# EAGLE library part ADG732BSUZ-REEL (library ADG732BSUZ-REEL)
16-/32-Channel, 4 , +1.8 V to +5.5 V and +/-2.5 V Analog Multiplexers. Source: Datasheet
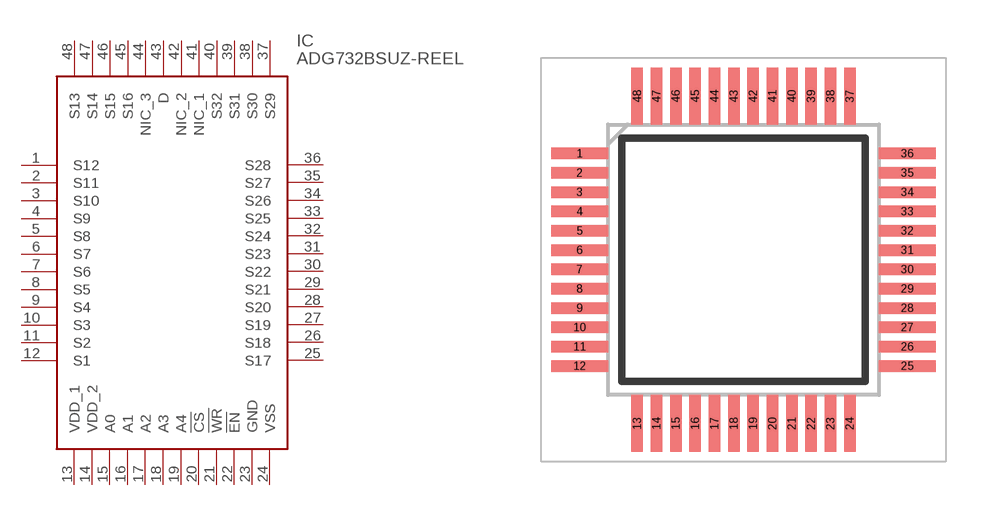
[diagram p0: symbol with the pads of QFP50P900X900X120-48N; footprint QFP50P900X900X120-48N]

Designator prefix IC

## ADG732BSUZ-REEL (Description: 16-/32-Channel, 4 , +1.8 V to +5.5 V and +/-2.5 V Analog Multiplexers.; Height: 1.2mm; Manufacturer_Name: Analog Devices; Manufacturer_Part_Number: ADG732BSUZ-REEL; Mouser_Part_Number: 584-ADG732BSUZ-R; Mouser_Price-Stock: https://www.mouser.co.uk/ProductDetail/Analog-Devices/ADG732BSUZ-REEL?qs=BpaRKvA4VqGYLEdHjoL3%2FQ%3D%3D)  [QFP50P900X900X120-48N]
1  S12
2  S11
3  S10
4  S9
5  S8
6  S7
7  S6
8  S5
9  S4
10  S3
11  S2
12  S1
13  VDD_1
14  VDD_2
15  A0
16  A1
17  A2
18  A3
19  A4
20  !CS
21  !WR
22  !EN
23  GND
24  VSS
25  S17
26  S18
27  S19
28  S20
29  S21
30  S22
31  S23
32  S24
33  S25
34  S26
35  S27
36  S28
37  S29
38  S30
39  S31
40  S32
41  NIC_1
42  NIC_2
43  D
44  NIC_3
45  S16
46  S15
47  S14
48  S13

## Footprint QFP50P900X900X120-48N (pad centres in mm)
SU-48 (TQFP)
smd 1.475 x 0.3: 1 -4.238,2.75; 2 -4.238,2.25; 3 -4.238,1.75; 4 -4.238,1.25; 5 -4.238,0.75; 6 -4.238,0.25; 7 -4.238,-0.25; 8 -4.238,-0.75; 9 -4.238,-1.25; 10 -4.238,-1.75; 11 -4.238,-2.25; 12 -4.238,-2.75; 25 4.238,-2.75; 26 4.238,-2.25; 27 4.238,-1.75; 28 4.238,-1.25; 29 4.238,-0.75; 30 4.238,-0.25; 31 4.238,0.25; 32 4.238,0.75; 33 4.238,1.25; 34 4.238,1.75; 35 4.238,2.25; 36 4.238,2.75
smd 0.3 x 1.475: 13 -2.75,-4.238; 14 -2.25,-4.238; 15 -1.75,-4.238; 16 -1.25,-4.238; 17 -0.75,-4.238; 18 -0.25,-4.238; 19 0.25,-4.238; 20 0.75,-4.238; 21 1.25,-4.238; 22 1.75,-4.238; 23 2.25,-4.238; 24 2.75,-4.238; 37 2.75,4.238; 38 2.25,4.238; 39 1.75,4.238; 40 1.25,4.238; 41 0.75,4.238; 42 0.25,4.238; 43 -0.25,4.238; 44 -0.75,4.238; 45 -1.25,4.238; 46 -1.75,4.238; 47 -2.25,4.238; 48 -2.75,4.238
